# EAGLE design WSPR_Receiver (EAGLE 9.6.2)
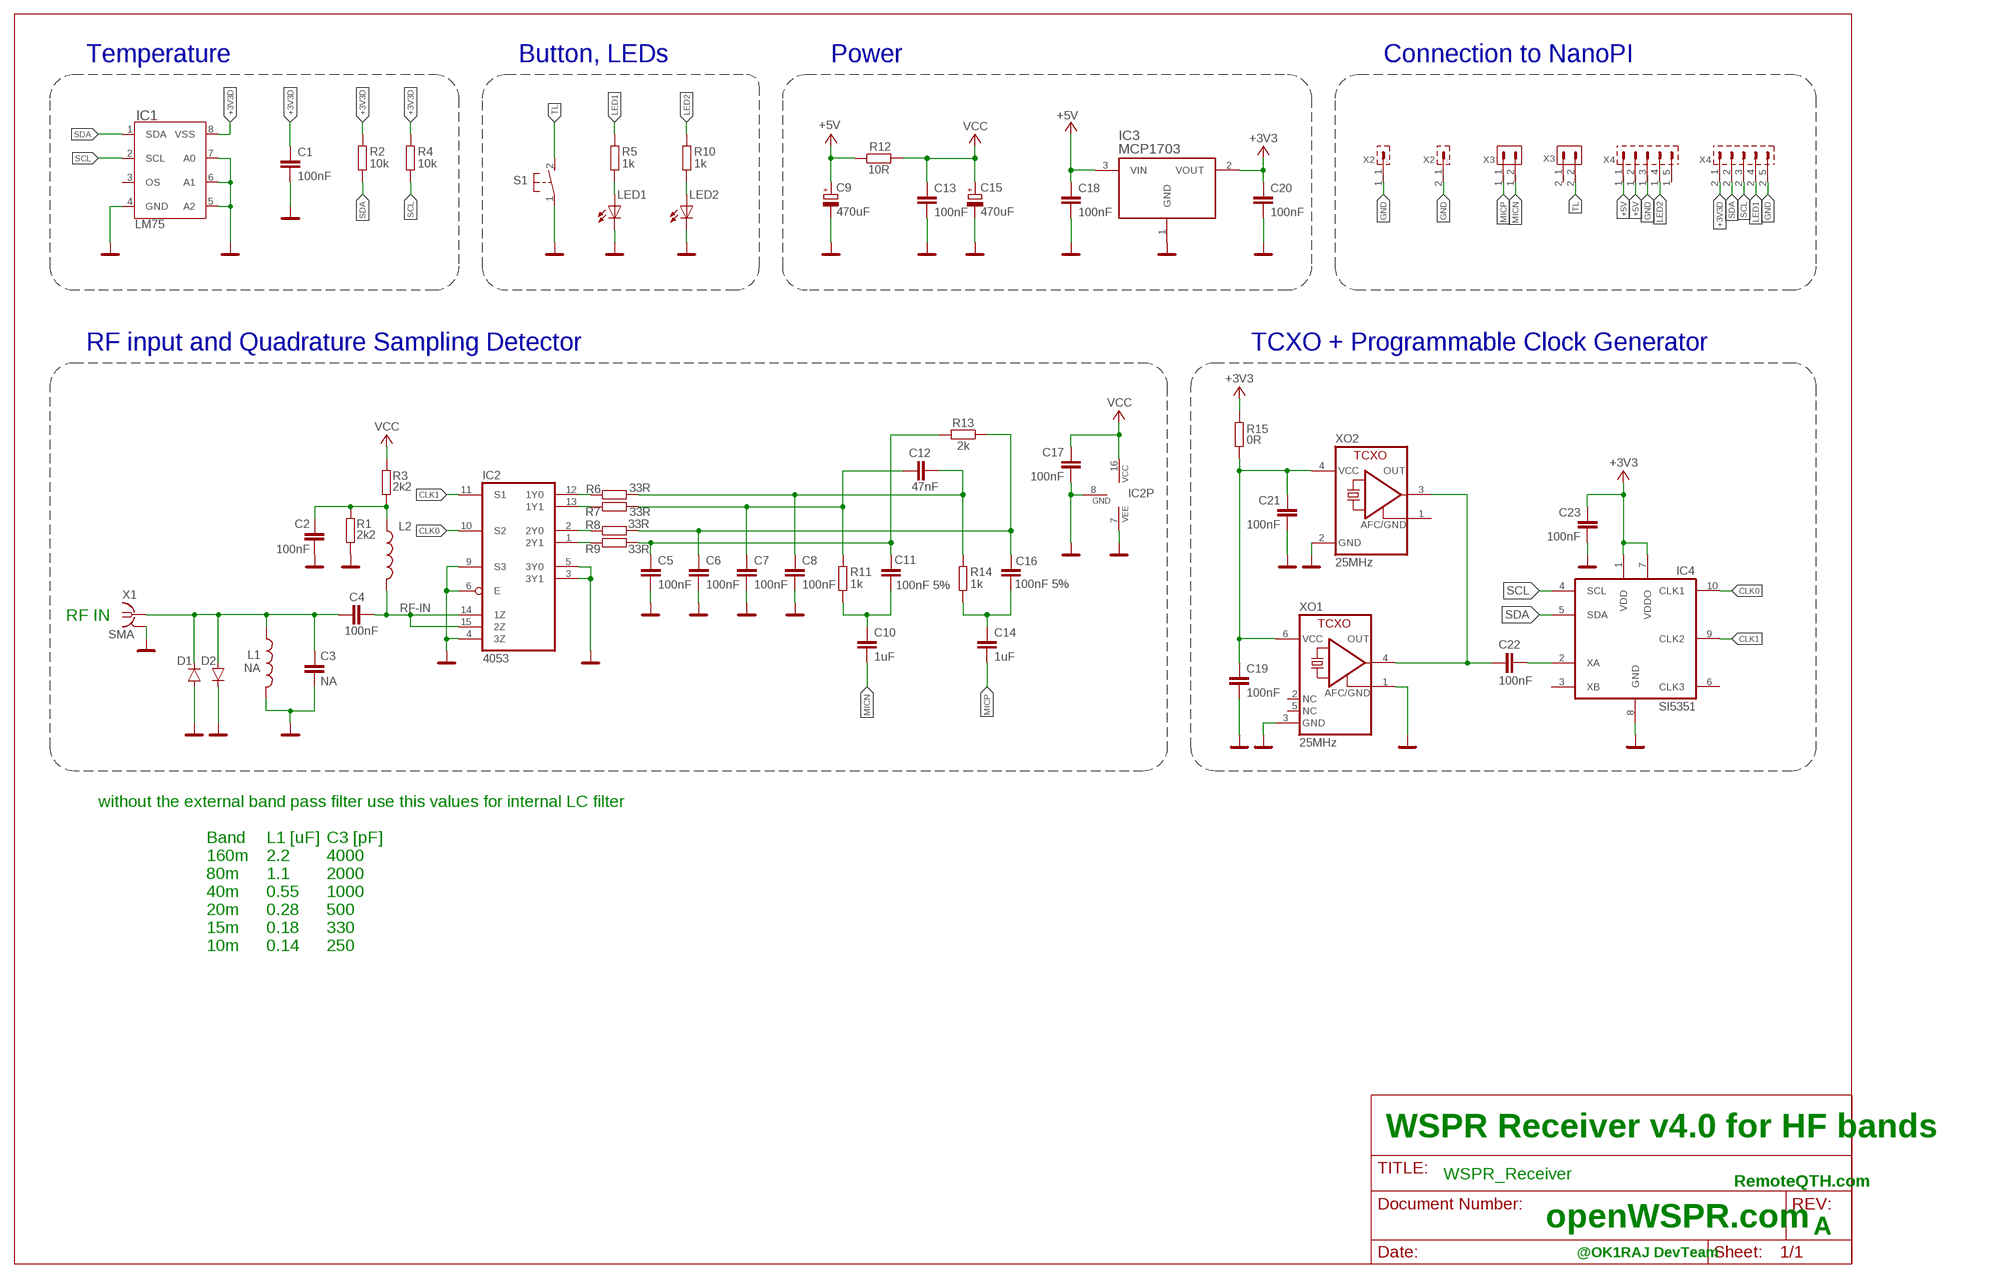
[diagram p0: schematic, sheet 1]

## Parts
C1  100nF  C-EUC0603  [C0603]
C2  100nF  C-EUC0603  [C0603]
C3  NA  C-EUC0805  [C0805]
C4  100nF  C-EUC0805  [C0805]
C5  100nF  C-EUC0603  [C0603]
C6  100nF  C-EUC0603  [C0603]
C7  100nF  C-EUC0603  [C0603]
C8  100nF  C-EUC0603  [C0603]
C9  470uF  CPOL-EUSMCD  [SMC_D]
C10  1uF  C-EUC0603  [C0603]
C11  100nF 5%  C-EUC0603  [C0603]
C12  47nF  C-EUC0603  [C0603]
C13  100nF  C-EUC0603  [C0603]
C14  1uF  C-EUC0603  [C0603]
C15  470uF  CPOL-EUSMCD  [SMC_D]
C16  100nF 5%  C-EUC0603  [C0603]
C17  100nF  C-EUC0603  [C0603]
C18  100nF  C-EUC0603  [C0603]
C19  100nF  C-EUC0603  [C0603]
C20  100nF  C-EUC0603  [C0603]
C21  100nF  C-EUC0603  [C0603]
C22  100nF  C-EUC0603  [C0603]
C23  100nF  C-EUC0603  [C0603]
D1  DIODE-MINIMELF  [MINIMELF]
D2  DIODE-MINIMELF  [MINIMELF]
IC1  LM75  [SOIC08]
IC2  4053  744053D  [SO16]
IC3  MCP1703  MCP1703T-5002E/CB  [SOT95P300X145-3N]
IC4  SI5351  SI5351A  [MSOP10]
L1  NA  L-USL1812  [L1812]
L2  INDUCTOR0805  [0805]
LED1  LEDL-934CB  [L-934CB]
LED2  LEDL-934CB  [L-934CB]
R1  2k2  R-EU_R0603  [R0603]
R2  10k  R-EU_R0603  [R0603]
R3  2k2  R-EU_R0603  [R0603]
R4  10k  R-EU_R0603  [R0603]
R5  1k  R-EU_R0603  [R0603]
R6  33R  R-EU_R0603  [R0603]
R7  33R  R-EU_R0603  [R0603]
R8  33R  R-EU_R0603  [R0603]
R9  33R  R-EU_R0603  [R0603]
R10  1k  R-EU_R0603  [R0603]
R11  1k  R-EU_R0603  [R0603]
R12  10R  R-EU_R0603  [R0603]
R13  2k  R-EU_R0603  [R0603]
R14  1k  R-EU_R0603  [R0603]
R15  0R  R-EU_R0603  [R0603]
S1  31-XX  [B3F-31XX]
X1  SMA  SMA-142-0711-821/826  [J502-ND-142-0711-821/826]
X2  S2G1_JUMP  [S2G1_JUM]
X3  S2G2_JUMP  [S2G2_JUM]
X4  S2G5_JUMP  [S2G5_JUM]
XO1  25MHz  7P-TCXO-25.000MHZ  [7P_OSCILATOR]
XO2  25MHz  TCXO-TG2520  [TG20_TCXO]

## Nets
1Y0: IC2.12(1Y0) R6.1
1Y1: IC2.13(1Y1) R7.1
2Y0: IC2.2(2Y0) R8.1
2Y1: IC2.1(2Y1) R9.1
25MHZ: C22.1 XO1.4(4-OUT) XO2.3(4-OUT)
27MHZ: C22.2 IC4.2(XA)
+3V3: C20.1 C23.1 IC3.2(VOUT) IC4.1(VDD) IC4.7(VDDO) R15.2
+3V3D: C1.1 IC1.8(VSS) R2.2 R4.2 X4.2_1
+5V: C9.+ C18.1 IC3.3(VIN) R12.1 X4.1_1 X4.1_2
CLK0: IC2.10(S2) IC4.10(CLK1)
CLK1: IC2.11(S1) IC4.9(CLK2)
GND: C1.2 C2.2 C3.1 C5.2 C6.2 C7.2 C8.2 C9.- C13.2 C15.- C17.2 C18.2 C19.2 C20.2 C21.2 C23.2 D1.A D2.C IC1.4(GND) IC1.5(A2) IC1.6(A1) IC1.7(A0) IC2.3(3Y1) IC2.4(3Z) IC2.5(3Y0) IC2.6(E) IC2.7(VEE) IC2.8(GND) IC2.9(S3) IC3.1(GND) IC4.8(GND) L1.2 LED1.-(C) LED2.-(C) R1.1 S1.1(P) X1.G@1 X1.G@2 X1.G@3 X1.G@4 X2.1_1 X2.2_1 X4.1_3 X4.2_5 XO1.1(1-AFC/GND) XO1.3(3-GND) XO2.2(3-GND)
LED1: R5.2 X4.2_4
LED2: R10.2 X4.1_4
MICN: C10.2 X3.1_2
MICP: C14.2 X3.1_1
N$7: C5.1 C11.1 R9.2 R13.2
N$8: C6.1 C16.1 R8.2 R13.1
N$9: C7.1 C12.1 R7.2 R11.2
N$10: C8.1 C12.2 R6.2 R14.2
N$11: C10.1 C11.2 R11.1
N$12: LED1.+(A) R5.1
N$13: C14.1 C16.2 R14.1
N$15: C2.1 L2.1 R1.2 R3.1
N$16: C3.2 C4.1 D1.C D2.A L1.1 X1.1
N$21: LED2.+(A) R10.1
RF-IN: C4.2 IC2.14(1Z) IC2.15(2Z) L2.2
SCL: IC1.2(SCL) IC4.4(SCL) R4.1 X4.2_3
SDA: IC1.1(SDA) IC4.5(SDA) R2.1 X4.2_2
TL: S1.2(S) X3.2_2
VCC: C13.1 C15.+ C17.1 IC2.16(VCC) R3.2 R12.2
VCC-RF1: C19.1 C21.1 R15.1 XO1.6(6-VCC) XO2.4(6-VCC)
Unconnected: IC1.3(OS) IC4.3(XB) IC4.6(CLK3) X3.2_1 X4.1_5 XO1.2(2-NC) XO1.5(5-NC) XO2.1(1-AFC/GND)

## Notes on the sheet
- Temperature | Button, LEDs | Power | Connection to NanoPI
- RF input and Quadrature Sampling Detector | TCXO + Programmable Clock Generator
- RF IN
- without the external band pass filter use this values for internal LC filter
- Band
  160m
  80m
  40m
  20m
  15m
  10m
- L1 [uF]
  2.2
  1.1
  0.55
  0.28
  0.18
  0.14
- C3 [pF]
  4000
  2000
  1000
  500
  330
  250
- WSPR Receiver v4.0 for HF bands
- RemoteQTH.com
- openWSPR.com
- A
- @OK1RAJ DevTeam

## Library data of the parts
C1-C8 C10-C14 C16-C18 C20 = rcl:C-EU: CAPACITOR, European symbol
C9 C15 = rcl:CPOL-EU: POLARIZED CAPACITOR, European symbol
C19 = rcl:C-EU: CAPACITOR, European symbol; LCSC_PART: N/A
C21 = resistor:C-EU: CAPACITOR, European symbol; LCSC_PART: C14663
C22 = resistor:C-EU: CAPACITOR, European symbol
C23 = rcl:C-EU: CAPACITOR, European symbol; LCSC_PART: C14663
D1 D2 = diode:DIODE-: DIODE
IC1 = #teplomery:LM75
IC2 = 74xx-eu:74*4053: Triple 2-channel analog multiplexer/demultiplexer Philips Semiconductor
IC3 = #Marek:MCP1703T-5002E/CB: Low Quiescent Current LDO Regulator; MPN: MCP1703T-5002E/CB; OC_FARNELL: 1439519; OC_NEWARK: 40M0640; PACKAGE: SOT-3; SUPPLIER: Microchip
IC4 = zelazko:SI5351
L1 = rcl:L-US: INDUCTOR, American symbol
L2 = adjacent-reality:INDUCTOR: Inductors
LED1 LED2 = #Marek:LED: LED
R1-R14 = rcl:R-EU_: RESISTOR, European symbol
R15 = rcl:R-EU_: RESISTOR, European symbol; LCSC_PART: C21189
S1 = switch-omron:31-XX: OMRON SWITCH; MPN: B3F-3100; OC_FARNELL: 959704; OC_NEWARK: 36M3582
X1 = con-coax:SMA-: SMA 50 Ohm End Launch Jack Receptacle - Round Contact; MF: JOHNSON COMPONENTS; MPN: 142-0711-821; OC_FARNELL: 1019328; OC_NEWARK: 16F3627
X2 = #PaJa_konektory:S2G1_JUMP: Radove konektory - koliky - dvojite - 2x1
X3 = #PaJa_konektory:S2G2_JUMP: Radove konektory - koliky - dvojite - 2x2
X4 = #PaJa_konektory:S2G5_JUMP: Radove konektory - koliky - dvojite - 2x5
XO1 = #my:7P-TCXO-25.000MHZ: TCXO
XO2 = #my:TCXO-TG2520

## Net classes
0 default: width 0.203 mm, drill 0.406 mm, clearance 0.203 mm

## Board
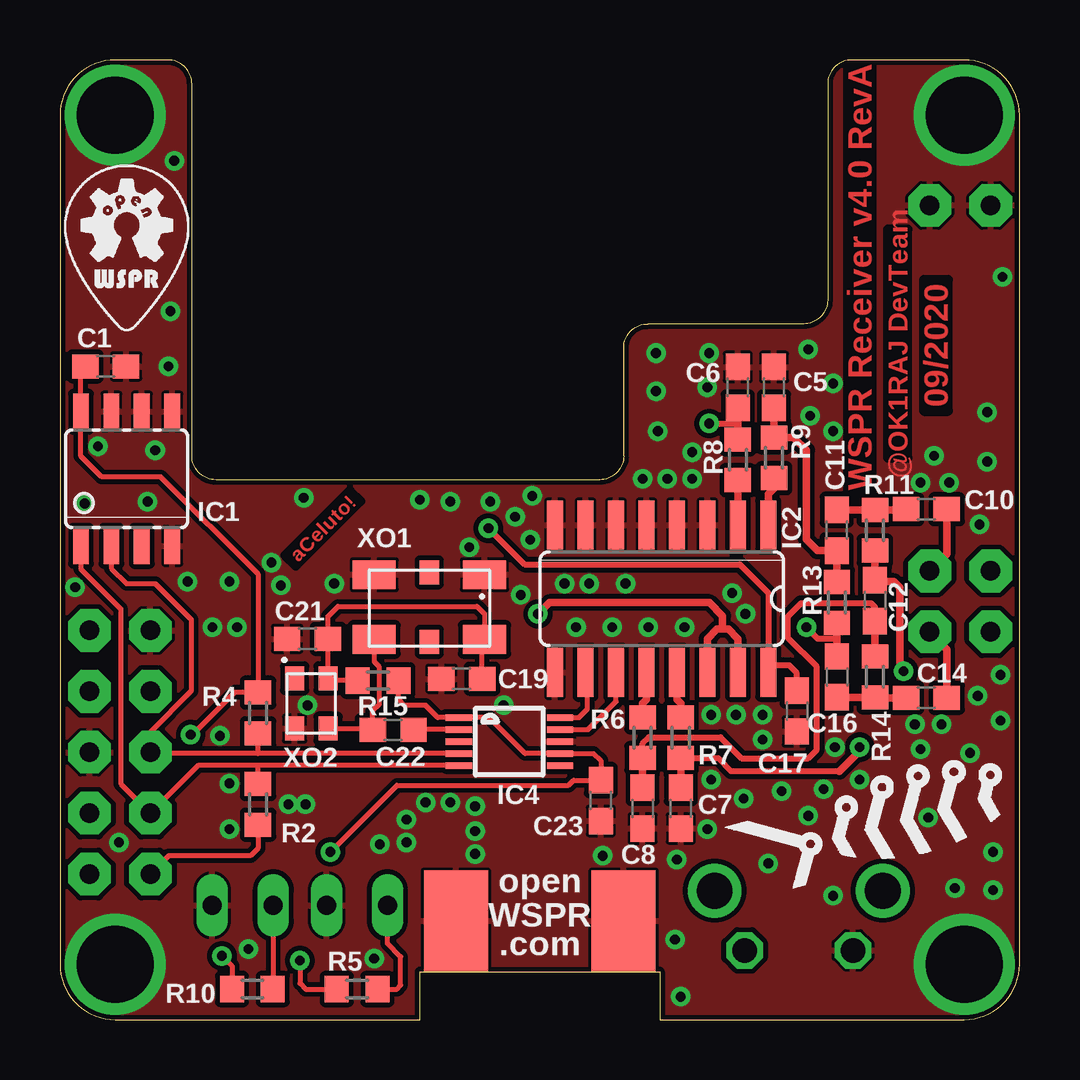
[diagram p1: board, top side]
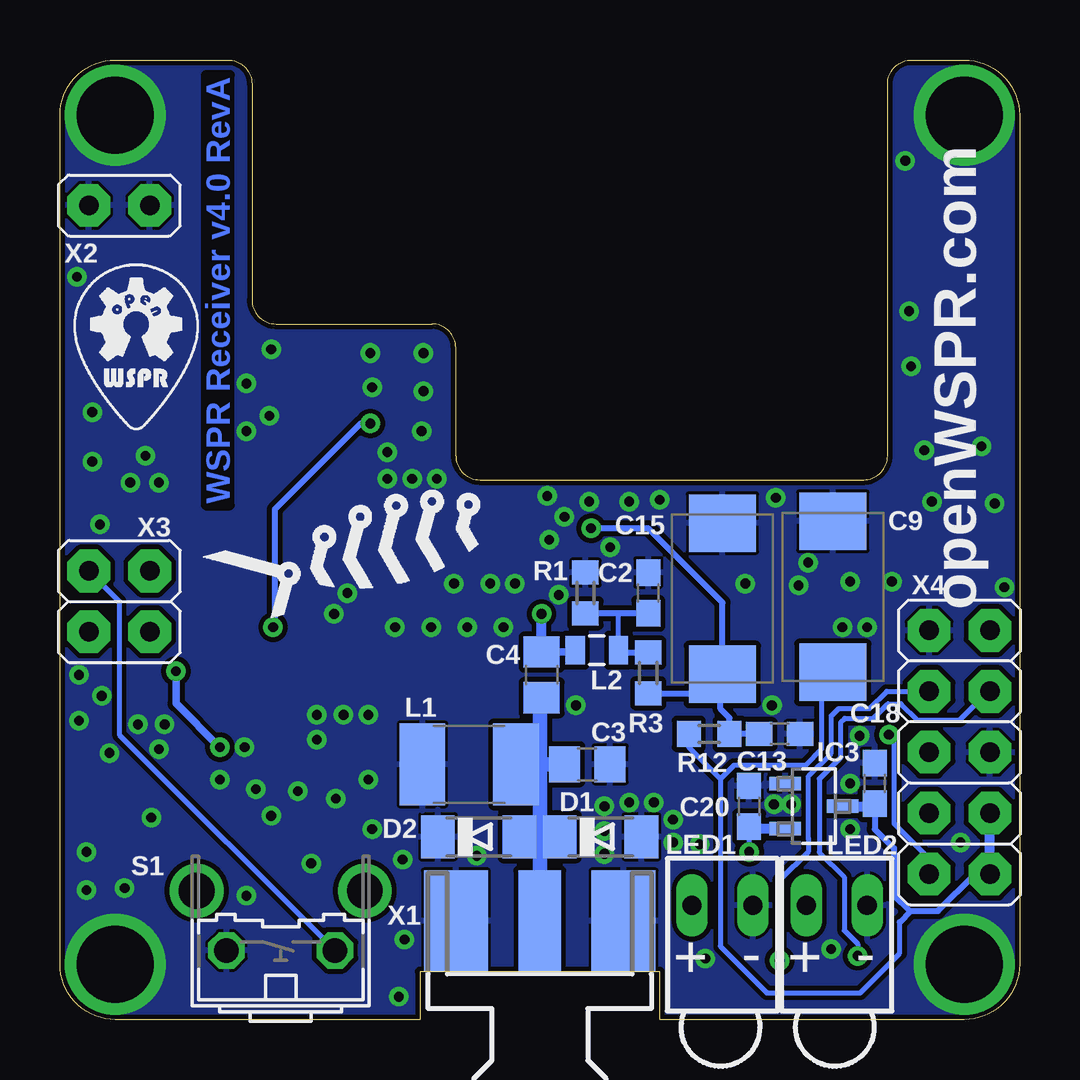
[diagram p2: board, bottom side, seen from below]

Size 40 x 40 mm. Coordinates in mm from the lower left corner, seen from the top.
Outline: 23.5,23.5 23.5,28 arc-90 24.5,29 31,29 arc90 32,30 32,39 arc-90 33,40 37.7,40 arc-90 40,37.7 40,2.3 arc-90 37.7,0 25,0 25,2 15,2 15,0 2.3,0 arc-90 0,2.3 0,37.7 arc-90 2.3,40 4.5,40 arc-90 5.5,39 5.5,23.5 arc90 6.5,22.5 22.5,22.5 arc90 23.5,23.5
Copper layers (1*16): Top 0.035mm / dielectric 1.6mm / Bottom 0.035mm
Design rules "JLCPCB_2layer_cheap *": minimum track width 5mil, minimum drill 0.2mm, track to track 5mil, track to pad 5mil, pad to pad 5mil, via to via 8mil, smd to smd 0mil, copper to edge 8mil, drill to drill 8mil, minimum pad ring 10mil, minimum via ring 8mil, stop-mask expansion 4mil, vias tented up to drill 0.7mm, thermal gap 5mil

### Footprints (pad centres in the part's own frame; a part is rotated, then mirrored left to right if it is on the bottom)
C0603 = smd 1.1 x 1: 1 -0.85,0; 2 0.85,0
C0805 = smd 1.3 x 1.5: 1 -0.95,0; 2 0.95,0
SMC_D = smd 2.4 x 2.8: + -3.15,0; - 3.15,0
MINIMELF = smd 1.4 x 1.8: A 1.7,0; C -1.7,0
SOIC08 = smd 0.66 x 1.5: 1 -1.905,-2.8; 2 -0.635,-2.8; 3 0.635,-2.8; 4 1.905,-2.8; 5 1.905,2.8; 6 0.635,2.8; 7 -0.635,2.8; 8 -1.905,2.8
SO16 = smd 0.66 x 2.032: 1 -4.445,-3.073; 2 -3.175,-3.073; 3 -1.905,-3.073; 4 -0.635,-3.073; 5 0.635,-3.073; 6 1.905,-3.073; 7 3.175,-3.073; 8 4.445,-3.073; 9 4.445,3.073; 10 3.175,3.073; 11 1.905,3.073; 12 0.635,3.073; 13 -0.635,3.073; 14 -1.905,3.073; 15 -3.175,3.073; 16 -4.445,3.073
SOT95P300X145-3N = smd 0.559 x 1.321: 1 -0.94,-1.194; 2 0.94,-1.194; 3 0,1.194
MSOP10 = smd 0.27 x 1.1: 1 -1,-2.113; 2 -0.5,-2.113; 3 0,-2.113; 4 0.5,-2.113; 5 1,-2.113; 6 1,2.113; 7 0.5,2.113; 8 0,2.113; 9 -0.5,2.113; 10 -1,2.113
L1812 = smd 1.9 x 3.4: 1 -1.95,0; 2 1.95,0
0805 = smd 0.8 x 1.2: 1 -0.9,0; 2 0.9,0
L-934CB = drill 0.8 long: + -1.27,0; - 1.27,0
R0603 = smd 1 x 1.1: 1 -0.85,0; 2 0.85,0
B3F-31XX = drill 1.016 octagon: 1 -2.261,-1.245; 2 2.261,-1.245 | drill 1.499 pad 2.159: 3 -3.505,1.245; 4 3.505,1.245
J502-ND-142-0711-821/826 = smd 4.191 x 1.778: 1 2.115,0 | smd 4.191 x 2.667: G@1 2.115,3.495; G@2 2.115,-3.495 | smd 4.191 x 2.667 bottom: G@3 2.115,3.495; G@4 2.115,-3.495
S2G1_JUM = drill 0.813 pad 1.778 octagon: 1_1 0,-1.27; 2_1 0,1.27
S2G2_JUM = drill 0.813 pad 1.778 octagon: 1_1 -1.27,-1.27; 1_2 1.27,-1.27; 2_1 -1.27,1.27; 2_2 1.27,1.27
S2G5_JUM = drill 0.813 pad 1.778 octagon: 1_1 -5.08,-1.27; 1_2 -2.54,-1.27; 1_3 0,-1.27; 1_4 2.54,-1.27; 1_5 5.08,-1.27; 2_1 -5.08,1.27; 2_2 -2.54,1.27; 2_3 0,1.27; 2_4 2.54,1.27; 2_5 5.08,1.27
7P_OSCILATOR = smd 1.8 x 1.2: 1 -2.3,-1.4; 3 2.3,-1.4; 4 2.3,1.3; 6 -2.3,1.3 | smd 0.8 x 1: 2 0,-1.5; 5 0,1.4
TG20_TCXO = smd 1 x 0.8: 1 -1.05,-0.7; 2 1.05,-0.7; 3 1.05,0.7; 4 -1.05,0.7

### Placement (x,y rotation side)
C1  1.91,27.23 0 top
C2  15.48,17.78 90 bottom
C3  18.02,10.64 180 bottom
C4  19.92,14.37 90 bottom
C5  29.77,26.35 90 top
C6  28.26,26.35 90 top
C7  25.88,8.81 270 top
C8  24.29,8.81 270 top
C9  7.78,17.62 90 bottom
C10  36.12,21.27 0 top
C11  32.38,20.4 90 top
C12  33.97,17.46 270 top
C13  10,11.91 0 bottom
C14  36.12,13.41 0 top
C15  12.38,17.54 90 bottom
C16  32.38,14.29 270 top
C17  30.72,12.86 270 top
C18  6.03,9.84 90 bottom
C19  16.75,14.21 180 top
C20  11.27,8.89 90 bottom
C21  10.32,15.88 180 top
C22  13.89,12.06 0 top
C23  22.54,9.13 270 top
D1  17.46,7.62 0 bottom
D2  22.54,7.62 0 bottom
IC1  2.78,22.54 0 top
IC2  25.08,17.54 180 top
IC3  8.57,8.89 270 bottom
IC4  18.73,11.59 270 top
L1  22.94,10.64 180 bottom
L2  17.62,15.4 180 bottom
LED1  12.38,4.76 0 bottom
LED2  7.62,4.76 0 bottom
R1  18.1,17.78 270 bottom
R2  8.26,8.97 270 top
R3  15.48,14.45 270 bottom
R4  8.26,12.78 90 top
R5  12.38,1.27 180 top
R6  24.29,11.75 270 top
R7  25.88,11.75 270 top
R8  28.26,23.34 90 top
R9  29.77,23.42 90 top
R10  8.02,1.27 180 top
R11  33.97,20.4 270 top
R12  12.94,11.91 0 bottom
R13  32.38,17.38 90 top
R14  33.97,14.29 90 top
R15  13.26,14.13 0 top
S1  30.8,4.13 0 bottom
U$1  [RYBICKA_12MM]  35.16,8.26 0 top
U$2  [RYBICKA_12MM]  26.59,19.53 0 bottom
U$3  [OPENWSPR-B_MEDIUM]  2.78,33.1 0 top
U$5  [OPENWSPR-B_MEDIUM]  36.83,28.97 0 bottom
X1  20,2 90 bottom
X2  37.53,33.94 90 bottom
X3  37.53,17.43 90 bottom
X4  2.5,11.14 90 bottom
XO1  15.4,17.14 180 top
XO2  10.48,13.18 270 top

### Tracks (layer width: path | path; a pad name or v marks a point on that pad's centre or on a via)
1Y0
  Top 0.305: IC2.12 24.45,13.34 24.29,13.18 R6.1
1Y1
  Top 0.305: IC2.13 25.72,13.34 25.88,13.18 R7.1
2Y0
  Top 0.305: R8.1 IC2.2
2Y1
  Top 0.305: R9.1 29.77,22.15 29.53,21.91 IC2.1
25MHZ
  Top 0.203: XO1.4 13.1,14.92 13.3,14.71 13.3,13.12 13.04,12.86 C22.1 12.98,12.13 XO2.3
27MHZ
  Top 0.203: IC4.2 14.76,12.09 C22.2
+3V3  (via drill 0.41)
  Top 0.203: R15.2 14.11,13.36 14.37,13.1 15.24,13.1 15.75,12.59 IC4.1 17.89,12.59 19.39,11.09 IC4.7 22.25,11.09 22.54,10.79 C23.1 21.41,9.98 21.19,9.76 14.05,9.76 v11.27,6.99
  Bottom 0.203: C20.1 v11.27,6.99
  Bottom 0.406: IC3.2 11.18,7.95 C20.1
+3V3D  (via drill 0.41)
  Top 0.203: 8.26,13.65 8.26,18.57 4.21,22.62 1.75,22.62 0.87,23.5 IC1.8 0.87,27.04 C1.1 | 8.26,13.65 R4.2 | R2.2 8.26,7.14 7.94,6.83 4.54,6.83 X4.2_1 | v5.45,11.88 5.53,11.88 7.3,13.65 8.26,13.65
  Bottom 0.203: X4.2_1 3.77,6.71 5.23,8.16 5.23,11.61 5.47,11.85 v5.45,11.88
+5V
  Bottom 0.203: R12.1 13.79,11.35 12.49,10.05 | 12.49,10.05 12.47,10.04 12.47,3.05 10.53,1.11 6.64,1.11 4.99,2.76 4.99,4.05 | C9.+ 8.26,13.99 8.26,11.27 8.93,10.6 11.9,10.6 12.44,10.05 12.49,10.05
  Bottom 0.254: C18.1 6.03,7.94 5.24,7.14 5.24,5.16 4.6,4.52 4.52,4.52 | 4.52,4.52 3.4,4.52 1.86,6.06 | 4.99,4.05 4.52,4.52
  Bottom 0.406: X4.1_2 X4.1_1 1.86,6.06 | IC3.3 6.13,8.89 C18.1
CLK0
  Top 0.203: IC4.10 21.64,12.59 21.99,12.94 21.99,14.39 IC2.10
CLK1
  Top 0.203: IC4.9 22.01,12.09 23.18,13.26 IC2.11
GND  (via drill 0.41, 3.2)
  other vias: 37.7,37.7 2.3,37.7 2.3,2.3 37.7,2.3 13.34,7.3 7.06,7.94 7.06,9.84 10.24,8.97 9.53,8.97 0.64,18.02 7.38,16.35 6.35,16.35 23.57,18.18 19.21,17.7 29.29,12.7 28.18,12.7 27.15,12.7 32.31,11.35 35.64,12.3 36.75,12.3 28.57,16.91 28.02,17.78 21.51,16.35 23.02,16.35 24.53,16.35 26.04,16.35 19.61,20 19.68,21.83 24.29,22.54 25.32,22.54 26.35,22.54 1.59,23.89 3.97,23.73 1.03,21.51 3.65,21.59 5.32,18.26 7.06,18.26 14.45,8.33 15.24,9.05 17.3,8.89 16.27,9.05 25.72,6.67 25.88,0.95 25.64,3.33 22.62,6.83 17.3,6.91 17.3,7.86 27.15,10 26.99,7.94 28.5,9.21 31.19,8.49 33.34,10 39.21,14.37 39.21,12.46 37.94,11.11 36.2,8.41 38.34,20.64 37.07,22.38 36.43,23.5 35.88,22.38 32.23,24.53 31.27,25.16 31.19,27.94 27.07,27.78 26.99,26.35 15,21.67 8.81,19.05 16.27,21.59 17.94,21.59 18.49,13.1 11.43,18.18 9.21,18.1 10.32,13.1 6.67,11.83 2.46,7.38 14.45,7.38 26.35,23.65 13.1,2.54 7.86,2.94 30.08,9.53 31.83,9.6 35.88,11.27 29.29,11.67 22.07,18.18 21.03,18.18 17.07,19.68 18.97,20.95 10.16,21.75 32.23,26.51 38.66,25.32 39.29,30.96 4.76,35.8 4.6,29.53 4.52,27.23 24.84,27.78 24.84,26.19 24.92,24.53 38.89,6.99 38.89,5.4 37.31,5.48 29.53,6.51 32.23,5.16 38.26,13.49 38.66,23.26
  pour Bottom: -0.64,40.32 40.96,40.32 40.96,-1.59 -0.64,-1.59
  pour Top: -0.64,40.48 41.2,40.48 41.2,-1.59 -0.64,-1.59
LED1  (via drill 0.41)
  Top 0.203: v10,2.46 10,1.51 10.24,1.27 R5.2
  Bottom 0.203: v10,2.46 10,5.79 8.81,6.99 8.81,7.54 8.8,7.54 8.8,10.15 7.85,11.1 7.85,12.66 7.54,12.97 6.25,12.97 5.54,13.68 X4.2_4
LED2  (via drill 0.41)
  Top 0.203: v6.75,2.65 7.17,2.23 R10.2
  Bottom 0.203: 2.5,12.49 1.31,13.68 X4.1_4 | v6.75,2.65 6.75,3.15 7.31,3.71 7.31,5.94 8.34,6.98 8.34,10.03 7.44,10.94 7.44,12.4 7.28,12.56 6.08,12.56 5.49,13.16 4.94,13.16 4.26,12.49 2.5,12.49 | 2.5,12.49
MICN
  Top 0.305: C10.2 36.97,19.41 X3.1_2
MICP
  Top 0.305: C14.2 36.97,15.42 36.26,16.13 X3.1_1
N$7
  Top 0.305: C5.1 R9.2 30.58,24.27 31.11,23.73 31.11,20 31.57,19.55 C11.1 R13.2
N$8  (via drill 0.41)
  Top 0.254: v31.11,16.35 31.59,15.88 32.38,15.88 | v27.07,24.84 28.18,24.84 28.26,24.77
  Top 0.305: R8.2 28.26,24.77 C6.1 | C16.1 32.38,15.88 R13.1
  Bottom 0.254: v31.11,16.35 31.04,16.43 31.04,21.27 27.46,24.84 v27.07,24.84
N$9  (via drill 0.41)
  Top 0.254: R7.2 27.44,10.9 27.99,10.35 32.5,10.35
  Top 0.305: R7.2 C7.1 | R11.2 C12.1 34.03,18.26 34.77,18.26 35,18.02 35,14.68 v35.16,14.53 | 32.5,10.35 33.34,11.19 v33.34,11.35
  Bottom 0.305: v35.16,14.53 35.16,13.18 v33.34,11.35
N$10
  Top 0.254: R6.2 24.29,11.51 24.55,11.77 27.54,11.77 28.41,10.89 31.2,10.89 31.55,11.24 31.55,14.71 30.35,15.91 30.35,16.8 30.9,17.36 33.8,17.36 33.97,17.19 C12.2
  Top 0.305: R6.2 C8.1 | R14.2 C12.2
N$11
  Top 0.305: C10.1 35.24,21.25 R11.1 C11.2
N$12
  Top 0.203: R5.1 14.05,1.27 14.21,1.43 14.21,2.62 13.65,3.17 LED1.+
N$13
  Top 0.305: C14.1 34,13.41 R14.1 C16.2
N$15
  Bottom 0.203: 16.75,16.93 16.75,15.43 L2.1
  Bottom 0.254: L2.1 16.62,15.3 R3.1 | C2.1 16.75,16.93 R1.2
N$16
  Bottom 0.61: X1.1 20,7.62 | 20,7.62 20,10.64 | 20,10.64 20,13.34 C4.1 | C3.2 20,10.64 | L1.1 20,10.64 | D1.C 20,7.62 | D2.A 20,7.62
N$21
  Top 0.203: LED2.+ 8.89,1.29 R10.1
RF-IN  (via drill 0.41)
  Top 0.305: IC2.14 26.99,15.88 27.38,16.27 27.62,16.27 | IC2.15 28.26,15.88 27.86,16.27 27.62,16.27 | 27.62,16.27 27.62,16.83 27.07,17.38 20.4,17.38 v19.92,16.91
  Bottom 0.305: C4.2 18.6,15.32 L2.2
  Bottom 0.406: C4.2 v19.92,16.91
SCL
  Top 0.203: 8.18,11.85 R4.1 8.26,11.09 | IC1.2 2.14,18.81 2.78,18.18 3.97,18.18 5.48,16.67 5.48,13.7 3.73,11.95 3.73,11.18 X4.2_3 3.82,11.09 8.26,11.09 | IC4.4 8.26,11.09
SDA
  Top 0.203: IC1.1 0.87,18.79 2.54,17.12 2.54,9.83 X4.2_2 5.76,10.59 8.26,10.59 | IC4.5 8.26,10.59 | R2.1 8.26,10.59
TL
  Bottom 0.203: S1.2 37.53,11.87 37.53,17.43 X3.2_2
VCC  (via drill 0.41)
  Top 0.254: v17.86,20.48 19.37,18.97 28.34,18.97 29.53,17.78 29.53,14.76 | 29.53,14.76 IC2.16 | 30.72,13.76 C17.1 30.72,14.45 30.4,14.76 29.53,14.76
  Bottom 0.203: 13.26,13.65 12.7,14.21 12.46,14.21
  Bottom 0.254: C13.1 R12.2 12.09,12.56 12.46,12.94 12.46,14.21 12.46,14.31 C15.+ 12.38,17.38 15.48,20.48 v17.86,20.48 | R3.2 13.31,13.6 13.26,13.65
VCC-RF1
  Top 0.203: R15.1 11.28,14.13 XO2.4 C21.1 11.17,16.8 11.59,17.22 17.38,17.22 17.7,16.91 XO1.6 17.6,15.74 C19.1

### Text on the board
Top: WSPR Receiver v4.0 RevA | @OK1RAJ DevTeam | 09/2020 | aCeluto!
Bottom: WSPR Receiver v4.0 RevA
tNames: open | WSPR | .com
bNames: openWSPR.com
